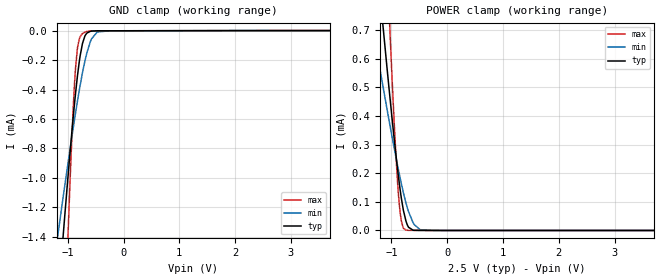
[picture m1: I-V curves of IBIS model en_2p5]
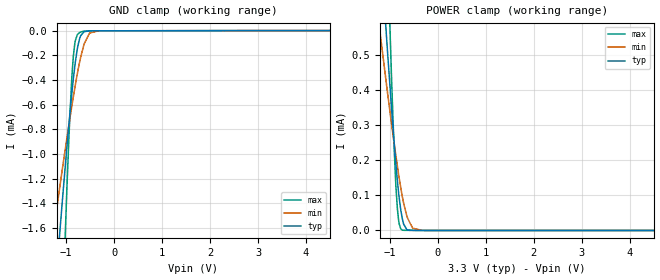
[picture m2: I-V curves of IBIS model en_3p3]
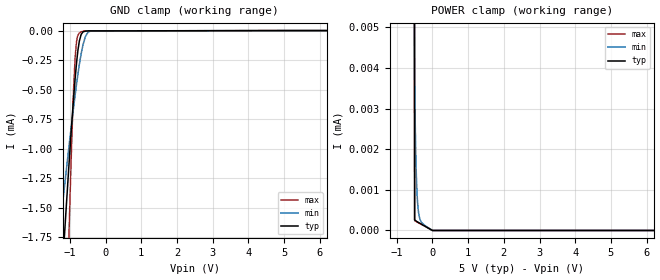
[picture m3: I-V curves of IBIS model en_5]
|Texas Instruments Incorporated
| High-Performance, 8000 VPK Reinforced Quad-Channel Digital Isolator
| Marketing part#   Digital Voltage Range   Package-type   #pins
| ISO7840FDW   2.25V-5.5V   SOIC   16
| ISO7840FDWW   2.25V-5.5V   SOIC   16
[IBIS Ver]   4.1
[File name]   iso7840f.ibs
[File Rev]   1.1
[Date]   5/11/2016
[Source]
| Texas Instruments Incorporated.
| Analog-eLab Design Center, HPA
| 12500 TI Blvd
| Dallas, TX -75243
[Notes]   Revision History:
| Rev 1.1: 5/11/2016
| - Add package component DWW
| Rev 1.0: 7/3/2015
| - Initial version of the model
| - Model generated from simulations in TISPICE
| - Model matched to SPICE simulation
| - C_comp although listed in numerical order of value are
|   obtained from varying PVT conditions. For PVT conditions for
|   each specific value refer the buffer description under
|   respective [Model]. IBIS model user is responsible for using
|   appropriate C_comp to simulate for Signal Integrity.
| - This is a relative part of ISO7841F.
|* EXCEPTION:   *
|* - For en_* models there will be leakage current in GROUND clamp  *
|*   because of a resistor(R0) connected to pad.   *
|* - For in_* models there will be leakage current in POWER clamp   *
|*   because of a resistor(R1) connected to pad.   *
[Disclaimer]
| This model is designed as an aid for customers of Texas Instruments.
| TI and its licensors and suppliers make no warranties, either expressed
| or implied, with respect to this  model, including the warranties of
| merchantability or fitness for a particular purpose. The model is
| provided solely on an "as is" basis. The entire risk as to its quality
| and performance is with the customer.
[Copyright]
(C) Copyright 2015 Texas Instruments Incorporated.All rights reserved.
|   ISO7840FDW
[Component]   ISO7840FDW
[Manufacturer]   TI
[Package]   |16 SOIC - DW package
|   typ   min   max
R_pkg   0.13558   0.12494   0.17928
L_pkg   2.10723nH   1.92454nH   2.85707nH
C_pkg   0.41633pF   0.21450pF   0.61276pF
[Pin]  signal_name   model_name   R_pin   L_pin   C_pin
1   VCC1   POWER   0.09703   2.25823nH  0.63889pF
2   GND1   GND   0.10567   2.15194nH  0.30706pF
3   INA   IN   0.12889   1.99554nH  0.21450pF
4   INB   IN   0.12623   1.94755nH  0.61276pF
5   INC   IN   0.12494   1.92646nH  0.36666pF
6   IND   IN   0.12883   1.99615nH  0.50841pF
7   NC   NC   0.17807   2.83638nH  0.45904pF
8   GND1   GND   0.08216   2.43955nH  0.44498pF
9   GND2   GND   0.10126   2.44074nH  0.40934pF
10   EN2   EN   0.17928   2.85707nH  0.52717pF
11   OUTD   OUT   0.14038   2.18765nH  0.43235pF
12   OUTC   OUT   0.12617   1.94399nH  0.32633pF
13   OUTB   OUT   0.12498   1.92454nH  0.37783pF
14   OUTA   OUT   0.14050   2.18615nH  0.38097pF
15   GND2   GND   0.08275   2.09014nH  0.75096pF
16   VCC2   POWER   0.09747   2.26909nH  0.67439pF
|   ISO7840FDWW
[Component]   ISO7840FDWW
[Manufacturer]   TI
[Package]   |16 SOIC - DWW package
|   typ   min   max
R_pkg   0.2986   0.2007   0.3729
L_pkg   6.1920nH   5.7068nH   6.9814nH
C_pkg   0.3776pF   0.0527pF   0.7658pF
[Pin]  signal_name   model_name   R_pin   L_pin   C_pin
1   VCC1   POWER   0.2515   6.9814nH   0.7658pF
2   GND1   GND   0.2414   6.4743nH   0.4827pF
3   INA   IN   0.3404   6.2419nH   0.3712pF
4   INB   IN   0.2997   5.8575nH   0.3661pF
5   INC   IN   0.3048   5.7068nH   0.3697pF
6   IND   IN   0.3229   5.9972nH   0.3885pF
7   NC   NC   0.3729   6.6301nH   0.3885pF
8   GND1   GND   0.2162   5.8346nH   0.4827pF
9   GND2   GND   0.2007   6.5823nH   0.5517pF
10   EN2   EN   0.3456   6.8632nH   0.3887pF
11   OUTD   OUT   0.3109   6.1891nH   0.3704pF
12   OUTC   OUT   0.2997   5.7473nH   0.3669pF
13   OUTB   OUT   0.3032   5.8251nH   0.3710pF
14   OUTA   OUT   0.3351   6.1684nH   0.0527pF
15   GND2   GND   0.2007   5.7509nH   0.5517pF
16   VCC2   POWER   0.2768   6.8945nH   0.0527pF
|   Model Selectors
[Model Selector] EN
en_2p5   2.5V digital Input
en_3p3   3.3V digital Input
en_5   5.0V digital Input
[Model Selector] IN
in_2p5   2.5V digital Input
in_3p3   3.3V digital Input
in_5   5.0V digital Input
[Model Selector] OUT
out_2p5   2.5V digital 3-state
out_3p3   3.3V digital 3-state
out_5   5.0V digital 3-state
| Models and submodels in the file (9): en_2p5 (Input), en_3p3 (Input), en_5 (Input), in_2p5 (Input), in_3p3 (Input), in_5 (Input), out_2p5 (3-state), out_3p3 (3-state), out_5 (3-state)
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|   en_2p5 Model
[Model]   en_2p5
Model_type   Input
Vinl = 0.75
Vinh = 1.75
|   typ   min   max
|   (nom PVT)   (fast PVT)   (slow PVT)
C_comp   3.303e-15   3.281e-15   1.151e-13
[Model spec]
|subparameter
Vinl   0.75   0.675   0.825
Vinh   1.75   1.575   1.925
| Where nom  PVT is Nominal Process, 2.5V, 27C
|   Fast PVT is Strong Process,  2.75V, -55C
|   Slow PVT is Weak Process,   2.25V, 150C
[Voltage Range]   2.5   2.25   2.75
|Junction Temperature
[Temperature Range]   27   150   -55
[Power Clamp Reference]   2.5   2.25   2.75
[GND Clamp Reference]   0   0   0
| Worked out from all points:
|   GND clamp passes 1 mA (typ) near -1.00 V on its own axis
|   POWER clamp passes 1 mA (typ) near -1.29 V on its own axis
[GND Clamp]
|   Voltage   I(typ)   I(min)   I(max)
-2.5V     -8.647mA   -5.195mA   -19.82mA
-1.224V   -2.083mA   -1.519mA   -3.979mA
-1.065V   -1.316mA   -1.086mA   -2.148mA
-1.001V   -1.021mA   -917uA     -1.46mA
-891.2mV  -548.7uA   -636.9uA   -451.9uA
-857.5mV  -419.8uA   -554.9uA   -246.1uA
-825.3mV  -308.5uA   -479.2uA   -120.6uA
-789.5mV  -203.1uA   -398.8uA   -52.86uA
-691mV    -36.17uA   -205.8uA   -10.4uA
-575mV    -3.575uA   -57.61uA   -2.24uA
-250mV    -1.373uA   -1.462uA   -1.451uA
5V        0A         0A         0A
[POWER Clamp]
|   Voltage   I(typ)   I(min)   I(max)
-2.5V     3.622mA    2.076mA    7.967mA
-1.351V   1.129mA    727.2uA    2.224mA
-1.196V   807.1uA    553.5uA    1.48mA
-1.053V   516.7uA    396.2uA    813.3uA
-990.2mV  394.3uA    329.2uA    537.7uA
-924.3mV  272.7uA    261.2uA    278.2uA
-874.8mV  189uA      212.4uA    126.7uA
-822.5mV  113uA      163.7uA    33.56uA
-740mV    33.03uA    96.34uA    1.225uA
-612.5mV  1.036uA    27.5uA     297.8nA
-486.3mV  250nA      2.81uA     235.3nA
5V        0A         0A         0A
|   en_3p3 Model
[Model]   en_3p3
Model_type   Input
Vinl = 0.99
Vinh = 2.31
|   typ   min   max
|   (nom PVT)   (fast PVT)   (slow PVT)
C_comp   3.303e-15   3.281e-15   1.158e-13
[Model spec]
|subparameter
Vinl   0.99   0.891   1.089
Vinh   2.31   2.079   2.541
| Where nom  PVT is Nominal Process, 3.3V, 27C
|   Fast PVT is Strong Process,  3.63V, -55C
|   Slow PVT is Weak Process,   2.97V, 150C
[Voltage Range]   3.3   2.97   3.63
|Junction Temperature
[Temperature Range]   27   150   -55
[Power Clamp Reference]   3.3   2.97   3.63
[GND Clamp Reference]   0   0   0
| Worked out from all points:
|   GND clamp passes 1 mA (typ) near -1.00 V on its own axis
|   POWER clamp passes 1 mA (typ) near -1.29 V on its own axis
[GND Clamp]
|   Voltage   I(typ)   I(min)   I(max)
-3.3V     -12.85mA   -7.552mA   -29.96mA
-1.251V   -2.215mA   -1.593mA   -4.295mA
-1.213V   -2.028mA   -1.488mA   -3.846mA
-1.063V   -1.305mA   -1.079mA   -2.122mA
-980.4mV  -927.6uA   -862.8uA   -1.246mA
-926mV    -691uA     -723.5uA   -729.1uA
-849.8mV  -392.1uA   -536.5uA   -209.7uA
-808.2mV  -255.7uA   -440.3uA   -80.89uA
-697.3mV  -41.71uA   -216.6uA   -11.76uA
-511.2mV  -2.293uA   -20.49uA   -2.098uA
-330mV    -1.815uA   -2.199uA   -1.916uA
6.6V      0A         0A         0A
[POWER Clamp]
|   Voltage   I(typ)   I(min)   I(max)
-3.3V     5.384mA    3.032mA    12.02mA
-1.242V   901.1uA    604.2uA    1.697mA
-1.198V   810uA      555uA      1.487mA
-1.049V   509.1uA    392uA      796uA
-965.9mV  348.5uA    303.8uA    437.1uA
-878.8mV  195.5uA    216.3uA    137uA
-842.5mV  140.2uA    181.9uA    60.64uA
-805.2mV  91.77uA    148.5uA    18.16uA
-737.2mV  31.27uA    94.34uA    1.112uA
-526mV    293.6nA    6.522uA    254.6nA
-330mV    164.9nA    232nA      159.7nA
6.6V      0A         0A         0A
|   en_5 Model
[Model]   en_5
Model_type   Input
Vinl = 1.5
Vinh = 3.5
|   typ   min   max
|   (nom PVT)   (fast PVT)   (slow PVT)
C_comp   3.303e-15   3.281e-15   1.164e-13
[Model spec]
|subparameter
Vinl   1.5   1.35   1.65
Vinh   3.5   3.15   3.85
| Where nom  PVT is Nominal Process, 5V, 27C
|   Fast PVT is Strong Process,  5.5V, -55C
|   Slow PVT is Weak Process,   4.5V, 150C
[Voltage Range]   5   4.5   5.5
|Junction Temperature
[Temperature Range]   27   150   -55
[Power Clamp Reference]   5   4.5   5.5
[GND Clamp Reference]   0   0   0
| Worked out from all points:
|   GND clamp passes 1 mA (typ) near -1.00 V on its own axis
[GND Clamp]
|   Voltage   I(typ)   I(min)   I(max)
-5V       -21.84mA   -12.59mA   -51.61mA
-1.304V   -2.48mA    -1.741mA   -4.932mA
-1.155V   -1.749mA   -1.331mA   -3.177mA
-1.128V   -1.616mA   -1.256mA   -2.86mA
-1.029V   -1.148mA   -990.1uA   -1.755mA
-927.5mV  -697.6uA   -727.4uA   -742.8uA
-855mV    -411.2uA   -549.1uA   -234.7uA
-790mV    -205uA     -400.1uA   -54.24uA
-685mV    -32.64uA   -196.1uA   -10.51uA
-567.5mV  -4.417uA   -52.27uA   -3.419uA
-369.5mV  -2.688uA   -3.564uA   -2.84uA
10V       0A         0A         0A
[POWER Clamp]
|   Voltage   I(typ)   I(min)   I(max)
-5V       371.1mA    133.7mA    611.2mA
-1.007V   426.4uA    346.8uA    609.2uA
-500mV    261.7nA    3.784uA    242nA
-491mV    253.9nA    3.115uA    237.6nA
-482mV    247nA      2.562uA    233.3nA
-473mV    240.7nA    2.107uA    228.9nA
-460mV    232.6nA    1.595uA    222.6nA
-432.5mV  217.1nA    909.5nA    209.3nA
-392mV    196.1nA    454.6nA    189.8nA
-306.5mV  153.2nA    197.5nA    148.4nA
-500uV    0A         0A         0A
10V       0A         0A         0A
